FUNCTION "Gest Asse B Boxing" : VOID
TITLE =Gestione Asse B Boxing Rotazione Polso +90Gr/0Gr/-90Gr
AUTHOR : MassimoZ
FAMILY : NovaSrl
VERSION : 0.1

BEGIN
NETWORK
TITLE ======== PACO 1 =======

NETWORK
TITLE =INS./DISIN.1
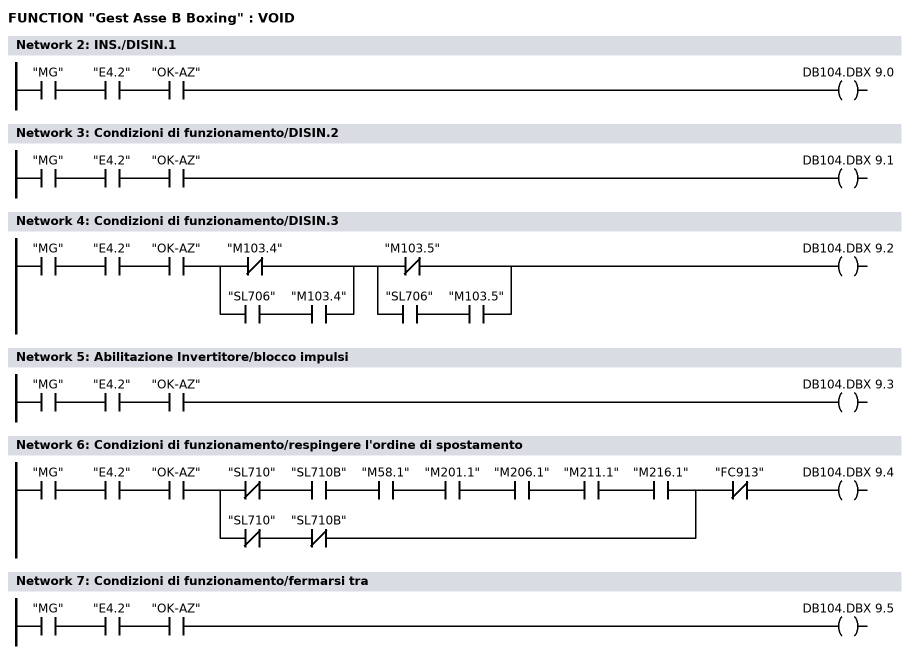
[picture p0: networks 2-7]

      U     "MG";
      U     "E4.2";
      U     "OK-AZ";
      =     DB104.DBX    9.0;
NETWORK
TITLE =Condizioni di funzionamento/DISIN.2

      U     "MG";
      U     "E4.2";
      U     "OK-AZ";
      =     DB104.DBX    9.1;
NETWORK
TITLE =Condizioni di funzionamento/DISIN.3

      U     "MG";
      U     "E4.2";
      U     "OK-AZ";
      U(    ;
      ON    "M103.4";
      O     ;
      U     "SL706";
      U     "M103.4";
      )     ;
      U(    ;
      ON    "M103.5";
      O     ;
      U     "SL706";
      U     "M103.5";
      )     ;
      =     DB104.DBX    9.2;
NETWORK
TITLE =Abilitazione Invertitore/blocco impulsi

      U     "MG";
      U     "E4.2";
      U     "OK-AZ";
      =     DB104.DBX    9.3;
NETWORK
TITLE =Condizioni di funzionamento/respingere l'ordine di spostamento

      U     "MG";
      U     "E4.2";
      U     "OK-AZ";
      U(    ;
      UN    "SL710";
      U     "SL710B";
      U     "M58.1";
      U     "M201.1";
      U     "M206.1";
      U     "M211.1";
      U     "M216.1";
      O     ;
      UN    "SL710";
      UN    "SL710B";
      )     ;
      UN    "FC913";
      =     DB104.DBX    9.4;
NETWORK
TITLE =Condizioni di funzionamento/fermarsi tra

      U     "MG";
      U     "E4.2";
      U     "OK-AZ";
      =     DB104.DBX    9.5;
NETWORK
TITLE =Attivare l'ordine di spostamento

      U(    ;
      U(    ;
      O     "M65.2";
      O     "M-ABPBS";
      O     "M+ABPBS";
      O     "M-ABPBD";
      O     "M+ABPBD";
      O     DB110.DBX    4.0;
      O     DB110.DBX    4.5;
      O     DB110.DBX    5.2;
      O     DB110.DBX    5.7;
      O     DB110.DBX    6.4;
      O     DB110.DBX    7.1;
      O     DB110.DBX   12.0;
      O     DB110.DBX   12.5;
      O     DB110.DBX   13.2;
      O     DB110.DBX   13.7;
      O     DB110.DBX   14.4;
      O     DB110.DBX   15.1;
      )     ;
      U(    ;
      UN    "SL710";
      U     "SL710B";
      O     ;
      UN    "SL710";
      UN    "SL710B";
      )     ;
      L     S5T#100MS;
      SE    T     52;
      NOP   0;
      NOP   0;
      NOP   0;
      U     T     52;
      )     ;
      FP    "M216.0";
      =     DB104.DBX    9.6;
NETWORK
TITLE =Reset memoria guasti
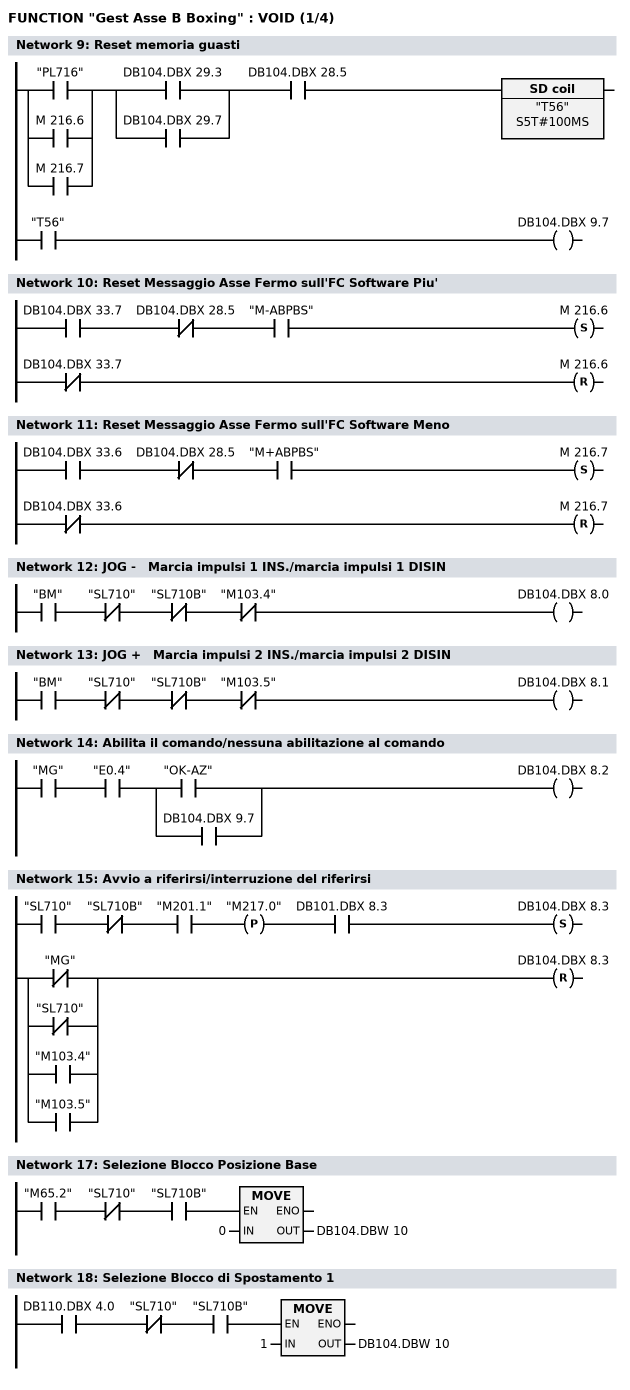
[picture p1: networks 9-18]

      U(    ;
      O     "PL716";
      O     M    216.6;
      O     M    216.7;
      )     ;
      U(    ;
      O     DB104.DBX   29.3;
      O     DB104.DBX   29.7;
      )     ;
      U     DB104.DBX   28.5;
      L     S5T#100MS;
      SE    "T56";
      NOP   0;
      NOP   0;
      NOP   0;
      U     "T56";
      =     DB104.DBX    9.7;
NETWORK
TITLE =Reset Messaggio Asse Fermo sull'FC Software Piu'

      U     DB104.DBX   33.7;
      UN    DB104.DBX   28.5;
      U     "M-ABPBS";
      S     M    216.6;
      UN    DB104.DBX   33.7;
      R     M    216.6;
      NOP   0;
NETWORK
TITLE =Reset Messaggio Asse Fermo sull'FC Software Meno

      U     DB104.DBX   33.6;
      UN    DB104.DBX   28.5;
      U     "M+ABPBS";
      S     M    216.7;
      UN    DB104.DBX   33.6;
      R     M    216.7;
      NOP   0;
NETWORK
TITLE =JOG -   Marcia impulsi 1 INS./marcia impulsi 1 DISIN

      U     "BM";
      UN    "SL710";
      UN    "SL710B";
      UN    "M103.4";
      =     DB104.DBX    8.0;
NETWORK
TITLE =JOG +   Marcia impulsi 2 INS./marcia impulsi 2 DISIN

      U     "BM";
      UN    "SL710";
      UN    "SL710B";
      UN    "M103.5";
      =     DB104.DBX    8.1;
NETWORK
TITLE =Abilita il comando/nessuna abilitazione al comando

      U     "MG";
      U     "E0.4";
      U(    ;
      O     "OK-AZ";
      O     DB104.DBX    9.7;
      )     ;
      =     DB104.DBX    8.2;
NETWORK
TITLE =Avvio a riferirsi/interruzione del riferirsi

      U     "SL710";
      UN    "SL710B";
      U     "M201.1";
      FP    "M217.0";
      U     DB101.DBX    8.3;
      S     DB104.DBX    8.3;
      U(    ;
      ON    "MG";
      ON    "SL710";
      O     "M103.4";
      O     "M103.5";
      )     ;
      R     DB104.DBX    8.3;
      NOP   0;
NETWORK
TITLE ======== SCELTA BLOCCO =======

NETWORK
TITLE =Selezione Blocco Posizione Base

      U     "M65.2";
      UN    "SL710";
      U     "SL710B";
      SPBNB _001;
      L     0;
      T     DB104.DBW   10;
_001: NOP   0;
NETWORK
TITLE =Selezione Blocco di Spostamento 1

      U     DB110.DBX    4.0;
      UN    "SL710";
      U     "SL710B";
      SPBNB _002;
      L     1;
      T     DB104.DBW   10;
_002: NOP   0;
NETWORK
TITLE =Selezione Blocco di Spostamento 2
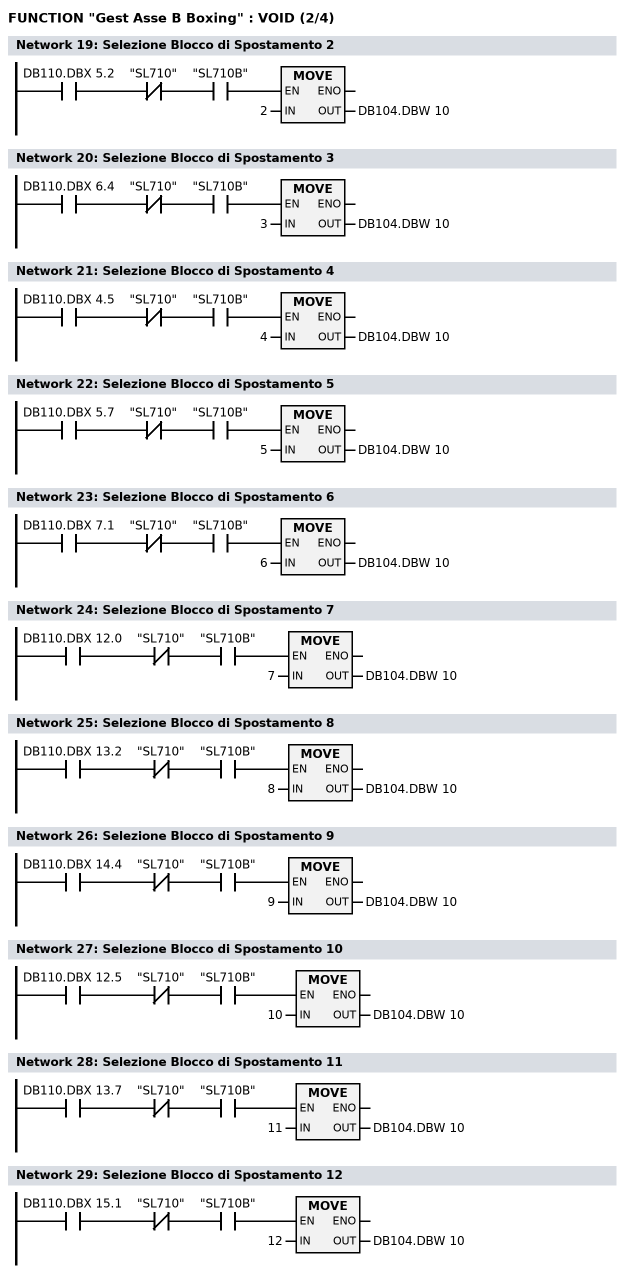
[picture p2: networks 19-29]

      U     DB110.DBX    5.2;
      UN    "SL710";
      U     "SL710B";
      SPBNB _003;
      L     2;
      T     DB104.DBW   10;
_003: NOP   0;
NETWORK
TITLE =Selezione Blocco di Spostamento 3

      U     DB110.DBX    6.4;
      UN    "SL710";
      U     "SL710B";
      SPBNB _004;
      L     3;
      T     DB104.DBW   10;
_004: NOP   0;
NETWORK
TITLE =Selezione Blocco di Spostamento 4

      U     DB110.DBX    4.5;
      UN    "SL710";
      U     "SL710B";
      SPBNB _005;
      L     4;
      T     DB104.DBW   10;
_005: NOP   0;
NETWORK
TITLE =Selezione Blocco di Spostamento 5

      U     DB110.DBX    5.7;
      UN    "SL710";
      U     "SL710B";
      SPBNB _006;
      L     5;
      T     DB104.DBW   10;
_006: NOP   0;
NETWORK
TITLE =Selezione Blocco di Spostamento 6

      U     DB110.DBX    7.1;
      UN    "SL710";
      U     "SL710B";
      SPBNB _007;
      L     6;
      T     DB104.DBW   10;
_007: NOP   0;
NETWORK
TITLE =Selezione Blocco di Spostamento 7

      U     DB110.DBX   12.0;
      UN    "SL710";
      U     "SL710B";
      SPBNB _008;
      L     7;
      T     DB104.DBW   10;
_008: NOP   0;
NETWORK
TITLE =Selezione Blocco di Spostamento 8

      U     DB110.DBX   13.2;
      UN    "SL710";
      U     "SL710B";
      SPBNB _009;
      L     8;
      T     DB104.DBW   10;
_009: NOP   0;
NETWORK
TITLE =Selezione Blocco di Spostamento 9

      U     DB110.DBX   14.4;
      UN    "SL710";
      U     "SL710B";
      SPBNB _00a;
      L     9;
      T     DB104.DBW   10;
_00a: NOP   0;
NETWORK
TITLE =Selezione Blocco di Spostamento 10

      U     DB110.DBX   12.5;
      UN    "SL710";
      U     "SL710B";
      SPBNB _00b;
      L     10;
      T     DB104.DBW   10;
_00b: NOP   0;
NETWORK
TITLE =Selezione Blocco di Spostamento 11

      U     DB110.DBX   13.7;
      UN    "SL710";
      U     "SL710B";
      SPBNB _00c;
      L     11;
      T     DB104.DBW   10;
_00c: NOP   0;
NETWORK
TITLE =Selezione Blocco di Spostamento 12

      U     DB110.DBX   15.1;
      UN    "SL710";
      U     "SL710B";
      SPBNB _00d;
      L     12;
      T     DB104.DBW   10;
_00d: NOP   0;
NETWORK
TITLE =Selezione Blocco di Spostamento 13 (0 Gradi Manuale)
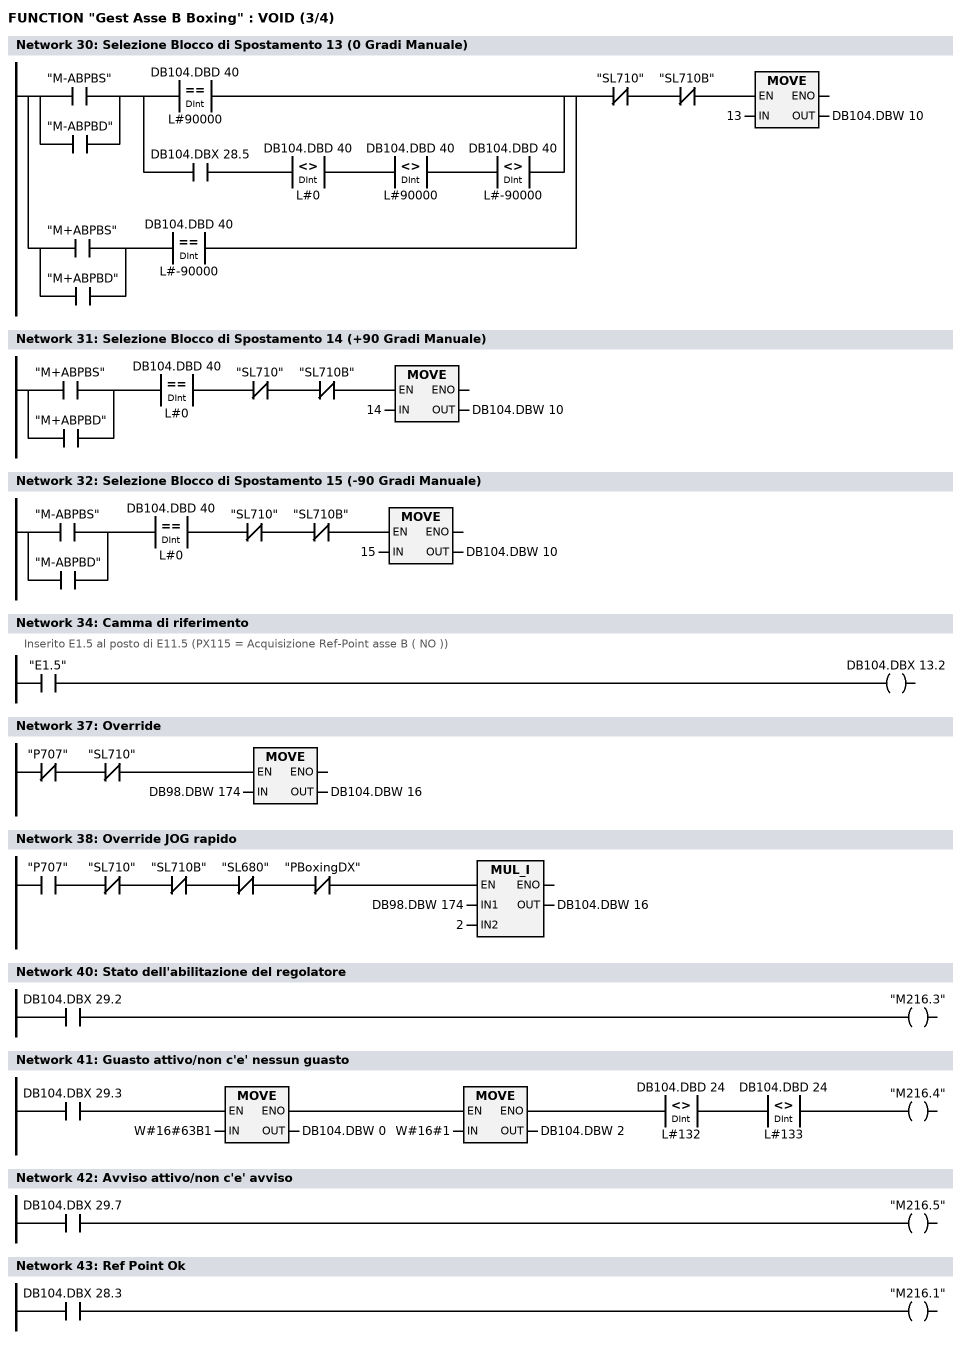
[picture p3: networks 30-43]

      U(    ;
      U(    ;
      O     "M-ABPBS";
      O     "M-ABPBD";
      )     ;
      U(    ;
      O(    ;
      L     DB104.DBD   40;
      L     L#90000;
      ==D   ;
      )     ;
      O     ;
      U     DB104.DBX   28.5;
      U(    ;
      L     DB104.DBD   40;
      L     L#0;
      <>D   ;
      )     ;
      U(    ;
      L     DB104.DBD   40;
      L     L#90000;
      <>D   ;
      )     ;
      U(    ;
      L     DB104.DBD   40;
      L     L#-90000;
      <>D   ;
      )     ;
      )     ;
      O     ;
      U(    ;
      O     "M+ABPBS";
      O     "M+ABPBD";
      )     ;
      U(    ;
      L     DB104.DBD   40;
      L     L#-90000;
      ==D   ;
      )     ;
      )     ;
      UN    "SL710";
      UN    "SL710B";
      SPBNB _00e;
      L     13;
      T     DB104.DBW   10;
_00e: NOP   0;
NETWORK
TITLE =Selezione Blocco di Spostamento 14 (+90 Gradi Manuale)

      U(    ;
      O     "M+ABPBS";
      O     "M+ABPBD";
      )     ;
      U(    ;
      L     DB104.DBD   40;
      L     L#0;
      ==D   ;
      )     ;
      UN    "SL710";
      UN    "SL710B";
      SPBNB _00f;
      L     14;
      T     DB104.DBW   10;
_00f: NOP   0;
NETWORK
TITLE =Selezione Blocco di Spostamento 15 (-90 Gradi Manuale)

      U(    ;
      O     "M-ABPBS";
      O     "M-ABPBD";
      )     ;
      U(    ;
      L     DB104.DBD   40;
      L     L#0;
      ==D   ;
      )     ;
      UN    "SL710";
      UN    "SL710B";
      SPBNB _010;
      L     15;
      T     DB104.DBW   10;
_010: NOP   0;
NETWORK
TITLE ======== POS PACO =======

NETWORK
TITLE =Camma di riferimento
//Inserito E1.5 al posto di E11.5 (PX115 = Acquisizione Ref-Point asse B ( NO ))
      U     "E1.5";
      =     DB104.DBX   13.2;
NETWORK
TITLE ======== PACO 2 ======= ( previsto )

NETWORK
TITLE ======== OVERRIDE ======

NETWORK
TITLE =Override

      UN    "P707";
      UN    "SL710";
      SPBNB _011;
      L     DB98.DBW  174;
      T     DB104.DBW   16;
_011: NOP   0;
NETWORK
TITLE =Override JOG rapido

      U     "P707";
      UN    "SL710";
      UN    "SL710B";
      UN    "SL680";
      UN    "PBoxingDX";
      SPBNB _012;
      L     DB98.DBW  174;
      L     2;
      *I    ;
      T     DB104.DBW   16;
_012: NOP   0;
NETWORK
TITLE ======== PAST 1 =======

NETWORK
TITLE =Stato dell'abilitazione del regolatore

      U     DB104.DBX   29.2;
      =     "M216.3";
NETWORK
TITLE =Guasto attivo/non c'e' nessun guasto

      U(    ;
      U(    ;
      U     DB104.DBX   29.3;
      SPBNB _013;
      L     W#16#63B1;
      T     DB104.DBW    0;
      SET   ;
      SAVE  ;
      CLR   ;
_013: U     BIE;
      )     ;
      SPBNB _014;
      L     W#16#1;
      T     DB104.DBW    2;
      SET   ;
      SAVE  ;
      CLR   ;
_014: U     BIE;
      )     ;
      U(    ;
      L     DB104.DBD   24;
      L     L#132;
      <>D   ;
      )     ;
      U(    ;
      L     DB104.DBD   24;
      L     L#133;
      <>D   ;
      )     ;
      =     "M216.4";
NETWORK
TITLE =Avviso attivo/non c'e' avviso

      U     DB104.DBX   29.7;
      =     "M216.5";
NETWORK
TITLE =Ref Point Ok

      U     DB104.DBX   28.3;
      =     "M216.1";
NETWORK
TITLE ======== POS PAST =======

NETWORK
TITLE ======== Lettura Quote =======

NETWORK
TITLE =Richiesta della Quota dell'asse B
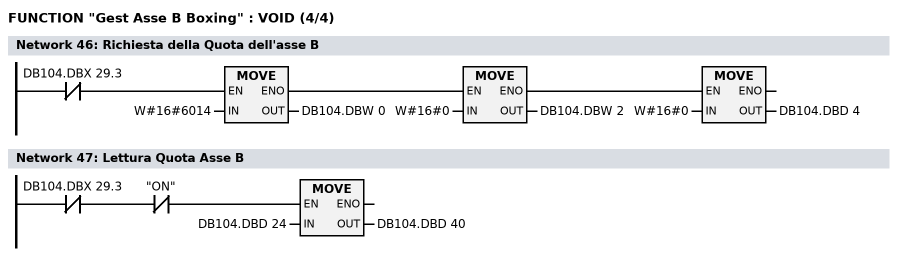
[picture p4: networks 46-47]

      U(    ;
      U(    ;
      UN    DB104.DBX   29.3;
      SPBNB _015;
      L     W#16#6014;
      T     DB104.DBW    0;
      SET   ;
      SAVE  ;
      CLR   ;
_015: U     BIE;
      )     ;
      SPBNB _016;
      L     W#16#0;
      T     DB104.DBW    2;
      SET   ;
      SAVE  ;
      CLR   ;
_016: U     BIE;
      )     ;
      SPBNB _017;
      L     W#16#0;
      T     DB104.DBD    4;
_017: NOP   0;
NETWORK
TITLE =Lettura Quota Asse B

      UN    DB104.DBX   29.3;
      UN    "ON";
      SPBNB _018;
      L     DB104.DBD   24;
      T     DB104.DBD   40;
_018: NOP   0;
NETWORK
TITLE ======== Caricamento quote sui Blocchi di Spostamento =======

NETWORK
TITLE =Caricamento Primo Posizionamento

      UN    "SL710";
      UN    "SL710B";
      U     DB99.DBX    3.3;
      O(    ;
      U     "MG";
      FP    M    254.4;
      )     ;
      O     "M219.0";
      =     L      0.0;
      U(    ;
      U(    ;
      U     L      0.0;
      UN    "M219.1";
      SPBNB _019;
      L     W#16#8051;
      T     DB104.DBW    0;
      SET   ;
      SAVE  ;
      CLR   ;
_019: U     BIE;
      )     ;
      SPBNB _01a;
      L     W#16#1;
      T     DB104.DBW    2;
      SET   ;
      SAVE  ;
      CLR   ;
_01a: U     BIE;
      )     ;
      SPBNB _01b;
      L     DB98.DBD  324;
      T     DB104.DBD    4;
_01b: NOP   0;
      U     L      0.0;
      BLD   102;
      S     "M219.0";
NETWORK
TITLE =Confronto Primo Posizionamento caricato nel 611U
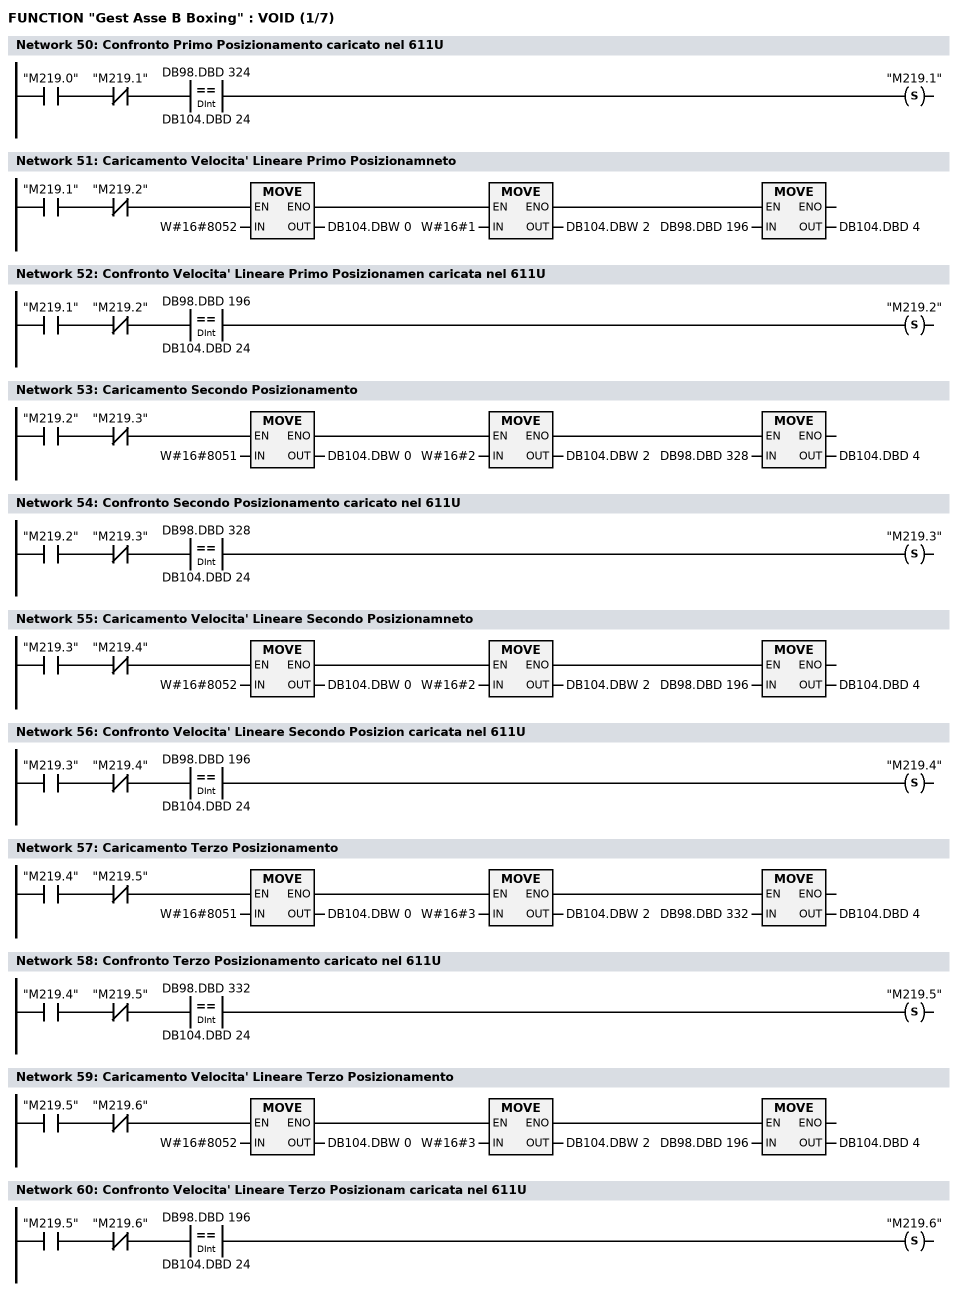
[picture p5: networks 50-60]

      U     "M219.0";
      UN    "M219.1";
      U(    ;
      L     DB98.DBD  324;
      L     DB104.DBD   24;
      ==D   ;
      )     ;
      S     "M219.1";
NETWORK
TITLE =Caricamento Velocita' Lineare Primo Posizionamneto

      U(    ;
      U(    ;
      U     "M219.1";
      UN    "M219.2";
      SPBNB _01c;
      L     W#16#8052;
      T     DB104.DBW    0;
      SET   ;
      SAVE  ;
      CLR   ;
_01c: U     BIE;
      )     ;
      SPBNB _01d;
      L     W#16#1;
      T     DB104.DBW    2;
      SET   ;
      SAVE  ;
      CLR   ;
_01d: U     BIE;
      )     ;
      SPBNB _01e;
      L     DB98.DBD  196;
      T     DB104.DBD    4;
_01e: NOP   0;
NETWORK
TITLE =Confronto Velocita' Lineare Primo Posizionamen caricata nel 611U

      U     "M219.1";
      UN    "M219.2";
      U(    ;
      L     DB98.DBD  196;
      L     DB104.DBD   24;
      ==D   ;
      )     ;
      S     "M219.2";
NETWORK
TITLE =Caricamento Secondo Posizionamento

      U(    ;
      U(    ;
      U     "M219.2";
      UN    "M219.3";
      SPBNB _01f;
      L     W#16#8051;
      T     DB104.DBW    0;
      SET   ;
      SAVE  ;
      CLR   ;
_01f: U     BIE;
      )     ;
      SPBNB _020;
      L     W#16#2;
      T     DB104.DBW    2;
      SET   ;
      SAVE  ;
      CLR   ;
_020: U     BIE;
      )     ;
      SPBNB _021;
      L     DB98.DBD  328;
      T     DB104.DBD    4;
_021: NOP   0;
NETWORK
TITLE =Confronto Secondo Posizionamento caricato nel 611U

      U     "M219.2";
      UN    "M219.3";
      U(    ;
      L     DB98.DBD  328;
      L     DB104.DBD   24;
      ==D   ;
      )     ;
      S     "M219.3";
NETWORK
TITLE =Caricamento Velocita' Lineare Secondo Posizionamneto

      U(    ;
      U(    ;
      U     "M219.3";
      UN    "M219.4";
      SPBNB _022;
      L     W#16#8052;
      T     DB104.DBW    0;
      SET   ;
      SAVE  ;
      CLR   ;
_022: U     BIE;
      )     ;
      SPBNB _023;
      L     W#16#2;
      T     DB104.DBW    2;
      SET   ;
      SAVE  ;
      CLR   ;
_023: U     BIE;
      )     ;
      SPBNB _024;
      L     DB98.DBD  196;
      T     DB104.DBD    4;
_024: NOP   0;
NETWORK
TITLE =Confronto Velocita' Lineare Secondo Posizion caricata nel 611U

      U     "M219.3";
      UN    "M219.4";
      U(    ;
      L     DB98.DBD  196;
      L     DB104.DBD   24;
      ==D   ;
      )     ;
      S     "M219.4";
NETWORK
TITLE =Caricamento Terzo Posizionamento

      U(    ;
      U(    ;
      U     "M219.4";
      UN    "M219.5";
      SPBNB _025;
      L     W#16#8051;
      T     DB104.DBW    0;
      SET   ;
      SAVE  ;
      CLR   ;
_025: U     BIE;
      )     ;
      SPBNB _026;
      L     W#16#3;
      T     DB104.DBW    2;
      SET   ;
      SAVE  ;
      CLR   ;
_026: U     BIE;
      )     ;
      SPBNB _027;
      L     DB98.DBD  332;
      T     DB104.DBD    4;
_027: NOP   0;
NETWORK
TITLE =Confronto Terzo Posizionamento caricato nel 611U

      U     "M219.4";
      UN    "M219.5";
      U(    ;
      L     DB98.DBD  332;
      L     DB104.DBD   24;
      ==D   ;
      )     ;
      S     "M219.5";
NETWORK
TITLE =Caricamento Velocita' Lineare Terzo Posizionamento

      U(    ;
      U(    ;
      U     "M219.5";
      UN    "M219.6";
      SPBNB _028;
      L     W#16#8052;
      T     DB104.DBW    0;
      SET   ;
      SAVE  ;
      CLR   ;
_028: U     BIE;
      )     ;
      SPBNB _029;
      L     W#16#3;
      T     DB104.DBW    2;
      SET   ;
      SAVE  ;
      CLR   ;
_029: U     BIE;
      )     ;
      SPBNB _02a;
      L     DB98.DBD  196;
      T     DB104.DBD    4;
_02a: NOP   0;
NETWORK
TITLE =Confronto Velocita' Lineare Terzo Posizionam caricata nel 611U

      U     "M219.5";
      UN    "M219.6";
      U(    ;
      L     DB98.DBD  196;
      L     DB104.DBD   24;
      ==D   ;
      )     ;
      S     "M219.6";
NETWORK
TITLE =Caricamento Quarto Posizionamento
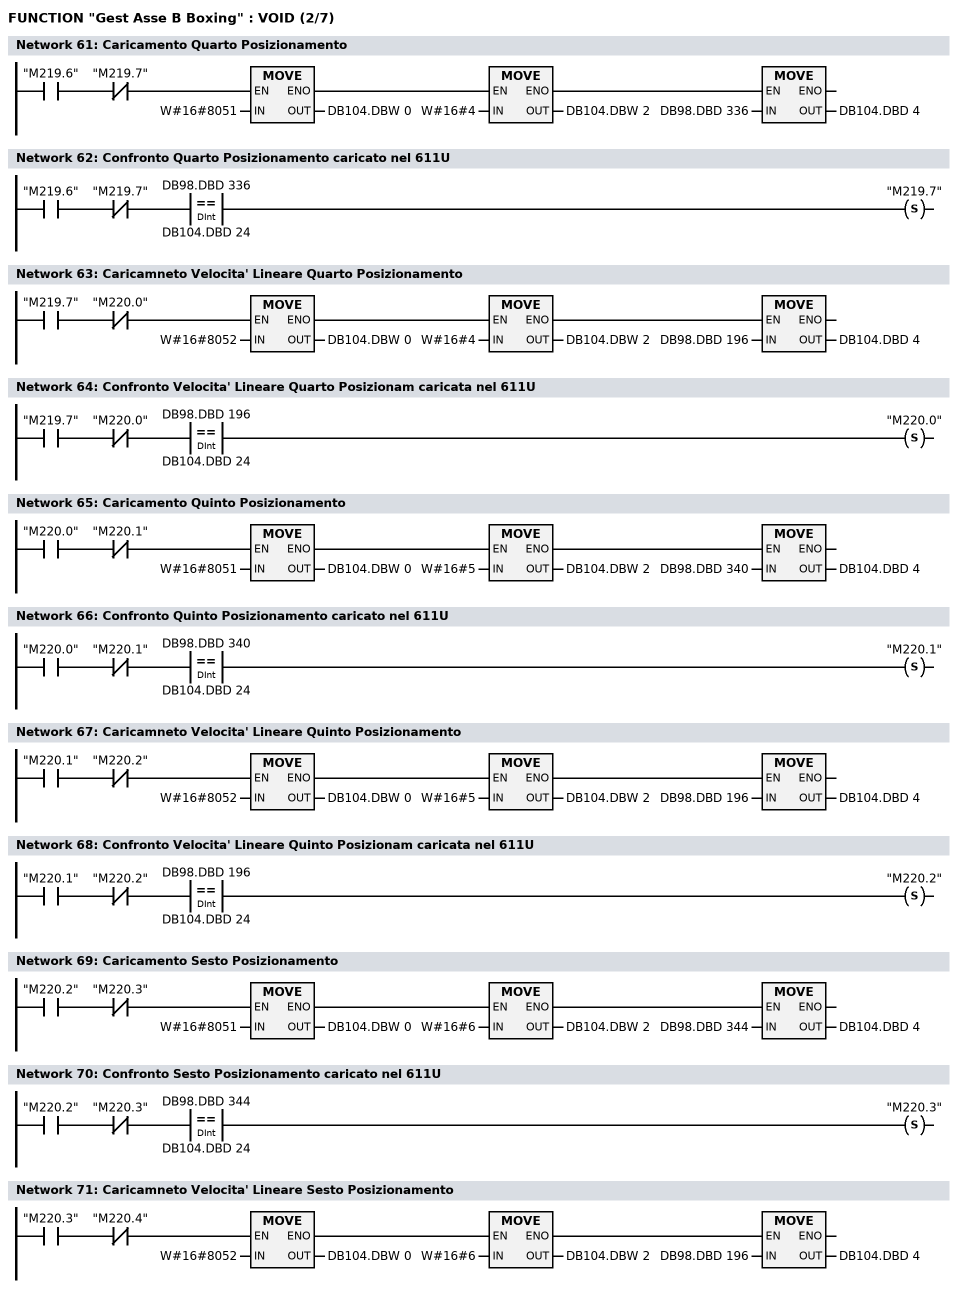
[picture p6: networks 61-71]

      U(    ;
      U(    ;
      U     "M219.6";
      UN    "M219.7";
      SPBNB _02b;
      L     W#16#8051;
      T     DB104.DBW    0;
      SET   ;
      SAVE  ;
      CLR   ;
_02b: U     BIE;
      )     ;
      SPBNB _02c;
      L     W#16#4;
      T     DB104.DBW    2;
      SET   ;
      SAVE  ;
      CLR   ;
_02c: U     BIE;
      )     ;
      SPBNB _02d;
      L     DB98.DBD  336;
      T     DB104.DBD    4;
_02d: NOP   0;
NETWORK
TITLE =Confronto Quarto Posizionamento caricato nel 611U

      U     "M219.6";
      UN    "M219.7";
      U(    ;
      L     DB98.DBD  336;
      L     DB104.DBD   24;
      ==D   ;
      )     ;
      S     "M219.7";
NETWORK
TITLE =Caricamneto Velocita' Lineare Quarto Posizionamento

      U(    ;
      U(    ;
      U     "M219.7";
      UN    "M220.0";
      SPBNB _02e;
      L     W#16#8052;
      T     DB104.DBW    0;
      SET   ;
      SAVE  ;
      CLR   ;
_02e: U     BIE;
      )     ;
      SPBNB _02f;
      L     W#16#4;
      T     DB104.DBW    2;
      SET   ;
      SAVE  ;
      CLR   ;
_02f: U     BIE;
      )     ;
      SPBNB _030;
      L     DB98.DBD  196;
      T     DB104.DBD    4;
_030: NOP   0;
NETWORK
TITLE =Confronto Velocita' Lineare Quarto Posizionam caricata nel 611U

      U     "M219.7";
      UN    "M220.0";
      U(    ;
      L     DB98.DBD  196;
      L     DB104.DBD   24;
      ==D   ;
      )     ;
      S     "M220.0";
NETWORK
TITLE =Caricamento Quinto Posizionamento

      U(    ;
      U(    ;
      U     "M220.0";
      UN    "M220.1";
      SPBNB _031;
      L     W#16#8051;
      T     DB104.DBW    0;
      SET   ;
      SAVE  ;
      CLR   ;
_031: U     BIE;
      )     ;
      SPBNB _032;
      L     W#16#5;
      T     DB104.DBW    2;
      SET   ;
      SAVE  ;
      CLR   ;
_032: U     BIE;
      )     ;
      SPBNB _033;
      L     DB98.DBD  340;
      T     DB104.DBD    4;
_033: NOP   0;
NETWORK
TITLE =Confronto Quinto Posizionamento caricato nel 611U

      U     "M220.0";
      UN    "M220.1";
      U(    ;
      L     DB98.DBD  340;
      L     DB104.DBD   24;
      ==D   ;
      )     ;
      S     "M220.1";
NETWORK
TITLE =Caricamneto Velocita' Lineare Quinto Posizionamento

      U(    ;
      U(    ;
      U     "M220.1";
      UN    "M220.2";
      SPBNB _034;
      L     W#16#8052;
      T     DB104.DBW    0;
      SET   ;
      SAVE  ;
      CLR   ;
_034: U     BIE;
      )     ;
      SPBNB _035;
      L     W#16#5;
      T     DB104.DBW    2;
      SET   ;
      SAVE  ;
      CLR   ;
_035: U     BIE;
      )     ;
      SPBNB _036;
      L     DB98.DBD  196;
      T     DB104.DBD    4;
_036: NOP   0;
NETWORK
TITLE =Confronto Velocita' Lineare Quinto Posizionam caricata nel 611U

      U     "M220.1";
      UN    "M220.2";
      U(    ;
      L     DB98.DBD  196;
      L     DB104.DBD   24;
      ==D   ;
      )     ;
      S     "M220.2";
NETWORK
TITLE =Caricamento Sesto Posizionamento

      U(    ;
      U(    ;
      U     "M220.2";
      UN    "M220.3";
      SPBNB _037;
      L     W#16#8051;
      T     DB104.DBW    0;
      SET   ;
      SAVE  ;
      CLR   ;
_037: U     BIE;
      )     ;
      SPBNB _038;
      L     W#16#6;
      T     DB104.DBW    2;
      SET   ;
      SAVE  ;
      CLR   ;
_038: U     BIE;
      )     ;
      SPBNB _039;
      L     DB98.DBD  344;
      T     DB104.DBD    4;
_039: NOP   0;
NETWORK
TITLE =Confronto Sesto Posizionamento caricato nel 611U

      U     "M220.2";
      UN    "M220.3";
      U(    ;
      L     DB98.DBD  344;
      L     DB104.DBD   24;
      ==D   ;
      )     ;
      S     "M220.3";
NETWORK
TITLE =Caricamneto Velocita' Lineare Sesto Posizionamento

      U(    ;
      U(    ;
      U     "M220.3";
      UN    "M220.4";
      SPBNB _03a;
      L     W#16#8052;
      T     DB104.DBW    0;
      SET   ;
      SAVE  ;
      CLR   ;
_03a: U     BIE;
      )     ;
      SPBNB _03b;
      L     W#16#6;
      T     DB104.DBW    2;
      SET   ;
      SAVE  ;
      CLR   ;
_03b: U     BIE;
      )     ;
      SPBNB _03c;
      L     DB98.DBD  196;
      T     DB104.DBD    4;
_03c: NOP   0;
NETWORK
TITLE =Confronto Velocita' Lineare Sesto Posizionam caricata nel 611U
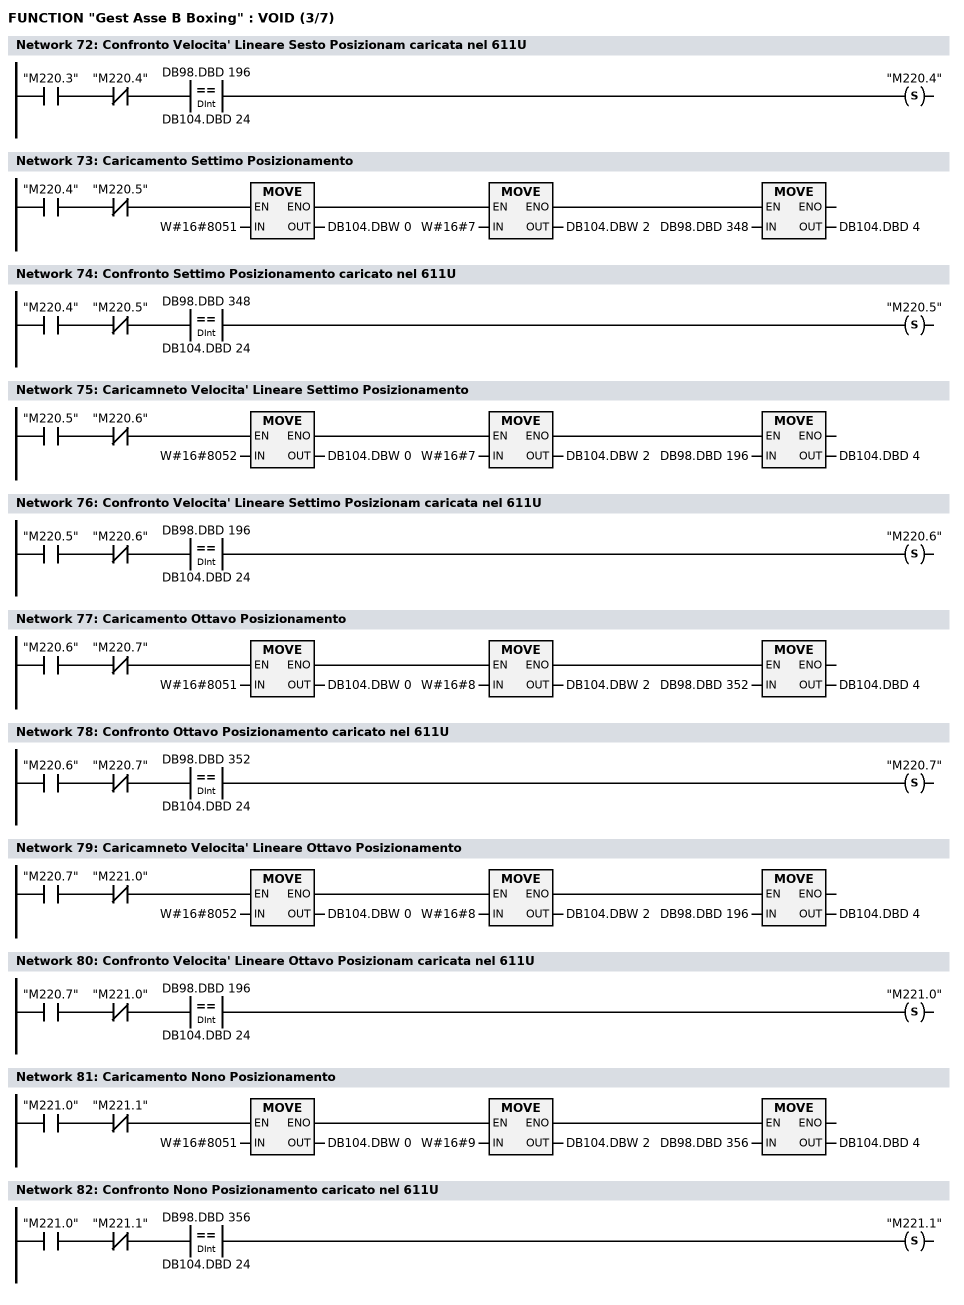
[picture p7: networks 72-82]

      U     "M220.3";
      UN    "M220.4";
      U(    ;
      L     DB98.DBD  196;
      L     DB104.DBD   24;
      ==D   ;
      )     ;
      S     "M220.4";
NETWORK
TITLE =Caricamento Settimo Posizionamento

      U(    ;
      U(    ;
      U     "M220.4";
      UN    "M220.5";
      SPBNB _03d;
      L     W#16#8051;
      T     DB104.DBW    0;
      SET   ;
      SAVE  ;
      CLR   ;
_03d: U     BIE;
      )     ;
      SPBNB _03e;
      L     W#16#7;
      T     DB104.DBW    2;
      SET   ;
      SAVE  ;
      CLR   ;
_03e: U     BIE;
      )     ;
      SPBNB _03f;
      L     DB98.DBD  348;
      T     DB104.DBD    4;
_03f: NOP   0;
NETWORK
TITLE =Confronto Settimo Posizionamento caricato nel 611U

      U     "M220.4";
      UN    "M220.5";
      U(    ;
      L     DB98.DBD  348;
      L     DB104.DBD   24;
      ==D   ;
      )     ;
      S     "M220.5";
NETWORK
TITLE =Caricamneto Velocita' Lineare Settimo Posizionamento

      U(    ;
      U(    ;
      U     "M220.5";
      UN    "M220.6";
      SPBNB _040;
      L     W#16#8052;
      T     DB104.DBW    0;
      SET   ;
      SAVE  ;
      CLR   ;
_040: U     BIE;
      )     ;
      SPBNB _041;
      L     W#16#7;
      T     DB104.DBW    2;
      SET   ;
      SAVE  ;
      CLR   ;
_041: U     BIE;
      )     ;
      SPBNB _042;
      L     DB98.DBD  196;
      T     DB104.DBD    4;
_042: NOP   0;
NETWORK
TITLE =Confronto Velocita' Lineare Settimo Posizionam caricata nel 611U

      U     "M220.5";
      UN    "M220.6";
      U(    ;
      L     DB98.DBD  196;
      L     DB104.DBD   24;
      ==D   ;
      )     ;
      S     "M220.6";
NETWORK
TITLE =Caricamento Ottavo Posizionamento

      U(    ;
      U(    ;
      U     "M220.6";
      UN    "M220.7";
      SPBNB _043;
      L     W#16#8051;
      T     DB104.DBW    0;
      SET   ;
      SAVE  ;
      CLR   ;
_043: U     BIE;
      )     ;
      SPBNB _044;
      L     W#16#8;
      T     DB104.DBW    2;
      SET   ;
      SAVE  ;
      CLR   ;
_044: U     BIE;
      )     ;
      SPBNB _045;
      L     DB98.DBD  352;
      T     DB104.DBD    4;
_045: NOP   0;
NETWORK
TITLE =Confronto Ottavo Posizionamento caricato nel 611U

      U     "M220.6";
      UN    "M220.7";
      U(    ;
      L     DB98.DBD  352;
      L     DB104.DBD   24;
      ==D   ;
      )     ;
      S     "M220.7";
NETWORK
TITLE =Caricamneto Velocita' Lineare Ottavo Posizionamento

      U(    ;
      U(    ;
      U     "M220.7";
      UN    "M221.0";
      SPBNB _046;
      L     W#16#8052;
      T     DB104.DBW    0;
      SET   ;
      SAVE  ;
      CLR   ;
_046: U     BIE;
      )     ;
      SPBNB _047;
      L     W#16#8;
      T     DB104.DBW    2;
      SET   ;
      SAVE  ;
      CLR   ;
_047: U     BIE;
      )     ;
      SPBNB _048;
      L     DB98.DBD  196;
      T     DB104.DBD    4;
_048: NOP   0;
NETWORK
TITLE =Confronto Velocita' Lineare Ottavo Posizionam caricata nel 611U

      U     "M220.7";
      UN    "M221.0";
      U(    ;
      L     DB98.DBD  196;
      L     DB104.DBD   24;
      ==D   ;
      )     ;
      S     "M221.0";
NETWORK
TITLE =Caricamento Nono Posizionamento

      U(    ;
      U(    ;
      U     "M221.0";
      UN    "M221.1";
      SPBNB _049;
      L     W#16#8051;
      T     DB104.DBW    0;
      SET   ;
      SAVE  ;
      CLR   ;
_049: U     BIE;
      )     ;
      SPBNB _04a;
      L     W#16#9;
      T     DB104.DBW    2;
      SET   ;
      SAVE  ;
      CLR   ;
_04a: U     BIE;
      )     ;
      SPBNB _04b;
      L     DB98.DBD  356;
      T     DB104.DBD    4;
_04b: NOP   0;
NETWORK
TITLE =Confronto Nono Posizionamento caricato nel 611U

      U     "M221.0";
      UN    "M221.1";
      U(    ;
      L     DB98.DBD  356;
      L     DB104.DBD   24;
      ==D   ;
      )     ;
      S     "M221.1";
NETWORK
TITLE =Caricamneto Velocita' Lineare Nono Posizionamento
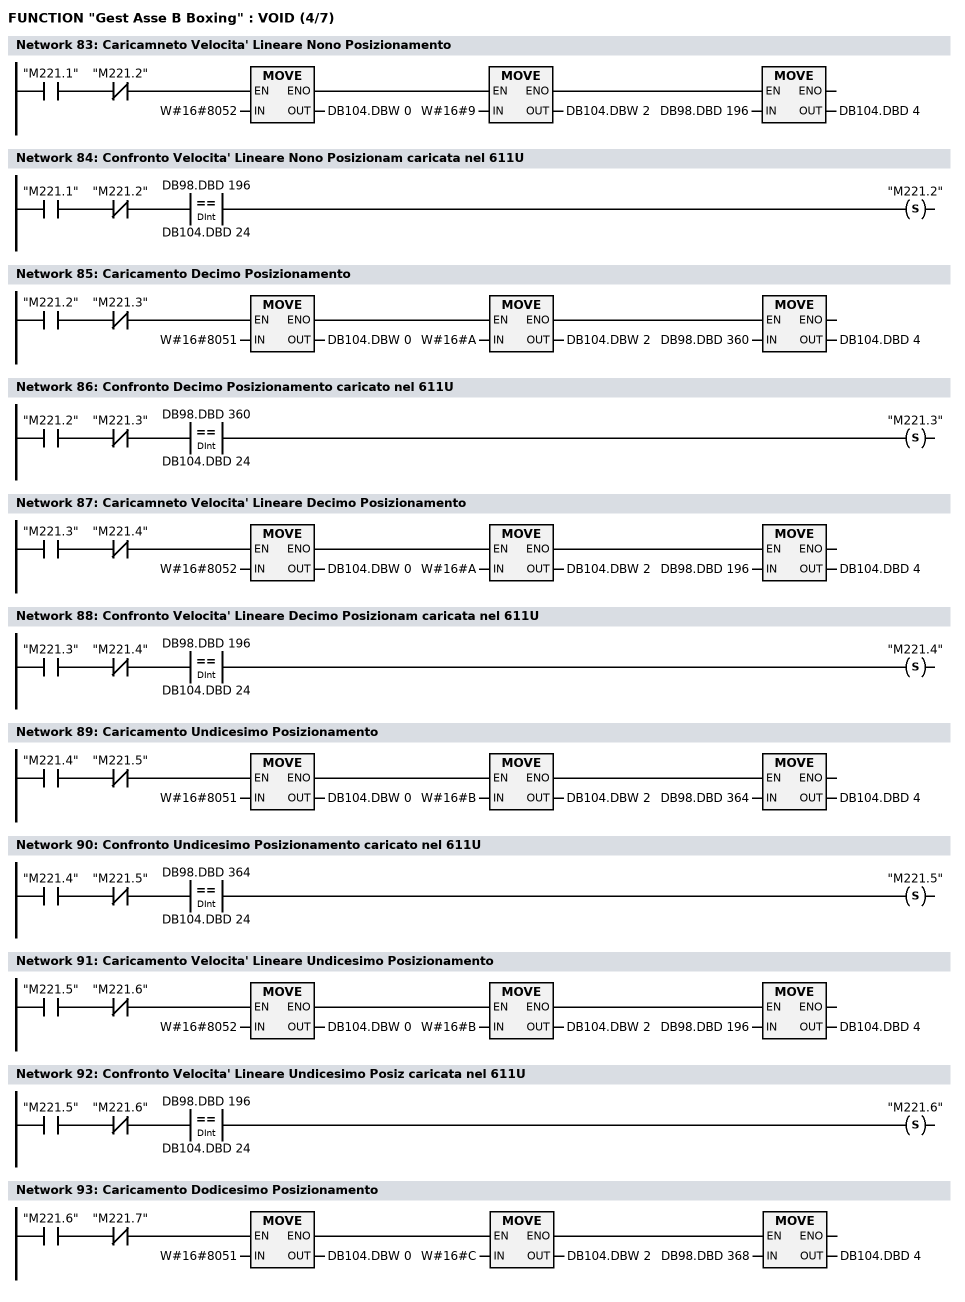
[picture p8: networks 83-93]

      U(    ;
      U(    ;
      U     "M221.1";
      UN    "M221.2";
      SPBNB _04c;
      L     W#16#8052;
      T     DB104.DBW    0;
      SET   ;
      SAVE  ;
      CLR   ;
_04c: U     BIE;
      )     ;
      SPBNB _04d;
      L     W#16#9;
      T     DB104.DBW    2;
      SET   ;
      SAVE  ;
      CLR   ;
_04d: U     BIE;
      )     ;
      SPBNB _04e;
      L     DB98.DBD  196;
      T     DB104.DBD    4;
_04e: NOP   0;
NETWORK
TITLE =Confronto Velocita' Lineare Nono Posizionam caricata nel 611U

      U     "M221.1";
      UN    "M221.2";
      U(    ;
      L     DB98.DBD  196;
      L     DB104.DBD   24;
      ==D   ;
      )     ;
      S     "M221.2";
NETWORK
TITLE =Caricamento Decimo Posizionamento

      U(    ;
      U(    ;
      U     "M221.2";
      UN    "M221.3";
      SPBNB _04f;
      L     W#16#8051;
      T     DB104.DBW    0;
      SET   ;
      SAVE  ;
      CLR   ;
_04f: U     BIE;
      )     ;
      SPBNB _050;
      L     W#16#A;
      T     DB104.DBW    2;
      SET   ;
      SAVE  ;
      CLR   ;
_050: U     BIE;
      )     ;
      SPBNB _051;
      L     DB98.DBD  360;
      T     DB104.DBD    4;
_051: NOP   0;
NETWORK
TITLE =Confronto Decimo Posizionamento caricato nel 611U

      U     "M221.2";
      UN    "M221.3";
      U(    ;
      L     DB98.DBD  360;
      L     DB104.DBD   24;
      ==D   ;
      )     ;
      S     "M221.3";
NETWORK
TITLE =Caricamneto Velocita' Lineare Decimo Posizionamento

      U(    ;
      U(    ;
      U     "M221.3";
      UN    "M221.4";
      SPBNB _052;
      L     W#16#8052;
      T     DB104.DBW    0;
      SET   ;
      SAVE  ;
      CLR   ;
_052: U     BIE;
      )     ;
      SPBNB _053;
      L     W#16#A;
      T     DB104.DBW    2;
      SET   ;
      SAVE  ;
      CLR   ;
_053: U     BIE;
      )     ;
      SPBNB _054;
      L     DB98.DBD  196;
      T     DB104.DBD    4;
_054: NOP   0;
NETWORK
TITLE =Confronto Velocita' Lineare Decimo Posizionam caricata nel 611U

      U     "M221.3";
      UN    "M221.4";
      U(    ;
      L     DB98.DBD  196;
      L     DB104.DBD   24;
      ==D   ;
      )     ;
      S     "M221.4";
NETWORK
TITLE =Caricamento Undicesimo Posizionamento

      U(    ;
      U(    ;
      U     "M221.4";
      UN    "M221.5";
      SPBNB _055;
      L     W#16#8051;
      T     DB104.DBW    0;
      SET   ;
      SAVE  ;
      CLR   ;
_055: U     BIE;
      )     ;
      SPBNB _056;
      L     W#16#B;
      T     DB104.DBW    2;
      SET   ;
      SAVE  ;
      CLR   ;
_056: U     BIE;
      )     ;
      SPBNB _057;
      L     DB98.DBD  364;
      T     DB104.DBD    4;
_057: NOP   0;
NETWORK
TITLE =Confronto Undicesimo Posizionamento caricato nel 611U

      U     "M221.4";
      UN    "M221.5";
      U(    ;
      L     DB98.DBD  364;
      L     DB104.DBD   24;
      ==D   ;
      )     ;
      S     "M221.5";
NETWORK
TITLE =Caricamento Velocita' Lineare Undicesimo Posizionamento

      U(    ;
      U(    ;
      U     "M221.5";
      UN    "M221.6";
      SPBNB _058;
      L     W#16#8052;
      T     DB104.DBW    0;
      SET   ;
      SAVE  ;
      CLR   ;
_058: U     BIE;
      )     ;
      SPBNB _059;
      L     W#16#B;
      T     DB104.DBW    2;
      SET   ;
      SAVE  ;
      CLR   ;
_059: U     BIE;
      )     ;
      SPBNB _05a;
      L     DB98.DBD  196;
      T     DB104.DBD    4;
_05a: NOP   0;
NETWORK
TITLE =Confronto Velocita' Lineare Undicesimo Posiz caricata nel 611U

      U     "M221.5";
      UN    "M221.6";
      U(    ;
      L     DB98.DBD  196;
      L     DB104.DBD   24;
      ==D   ;
      )     ;
      S     "M221.6";
NETWORK
TITLE =Caricamento Dodicesimo Posizionamento

      U(    ;
      U(    ;
      U     "M221.6";
      UN    "M221.7";
      SPBNB _05b;
      L     W#16#8051;
      T     DB104.DBW    0;
      SET   ;
      SAVE  ;
      CLR   ;
_05b: U     BIE;
      )     ;
      SPBNB _05c;
      L     W#16#C;
      T     DB104.DBW    2;
      SET   ;
      SAVE  ;
      CLR   ;
_05c: U     BIE;
      )     ;
      SPBNB _05d;
      L     DB98.DBD  368;
      T     DB104.DBD    4;
_05d: NOP   0;
NETWORK
TITLE =Confronto Dodicesimo Posizionamento caricato nel 611U
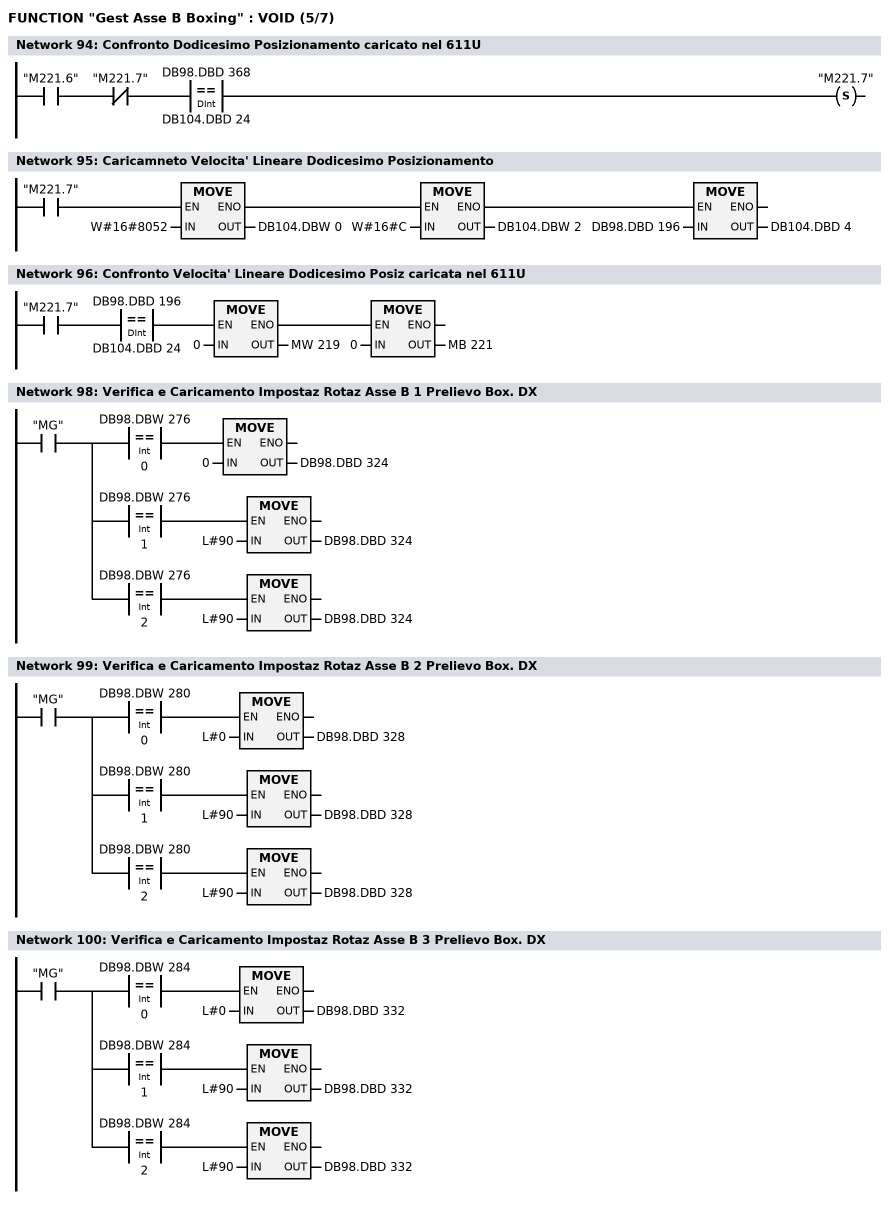
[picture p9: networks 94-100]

      U     "M221.6";
      UN    "M221.7";
      U(    ;
      L     DB98.DBD  368;
      L     DB104.DBD   24;
      ==D   ;
      )     ;
      S     "M221.7";
NETWORK
TITLE =Caricamneto Velocita' Lineare Dodicesimo Posizionamento

      U(    ;
      U(    ;
      U     "M221.7";
      SPBNB _05e;
      L     W#16#8052;
      T     DB104.DBW    0;
      SET   ;
      SAVE  ;
      CLR   ;
_05e: U     BIE;
      )     ;
      SPBNB _05f;
      L     W#16#C;
      T     DB104.DBW    2;
      SET   ;
      SAVE  ;
      CLR   ;
_05f: U     BIE;
      )     ;
      SPBNB _060;
      L     DB98.DBD  196;
      T     DB104.DBD    4;
_060: NOP   0;
NETWORK
TITLE =Confronto Velocita' Lineare Dodicesimo Posiz caricata nel 611U

      U(    ;
      U     "M221.7";
      U(    ;
      L     DB98.DBD  196;
      L     DB104.DBD   24;
      ==D   ;
      )     ;
      SPBNB _061;
      L     0;
      T     MW   219;
      SET   ;
      SAVE  ;
      CLR   ;
_061: U     BIE;
      )     ;
      SPBNB _062;
      L     0;
      T     MB   221;
_062: NOP   0;
NETWORK
TITLE ======== Caricamento Softkey OP sulle DB delle Quote Asse B =====

NETWORK
TITLE =Verifica e Caricamento Impostaz Rotaz Asse B 1 Prelievo Box. DX

      U     "MG";
      =     L      0.0;
      U     L      0.0;
      U(    ;
      L     DB98.DBW  276;
      L     0;
      ==I   ;
      )     ;
      SPBNB _063;
      L     0;
      T     DB98.DBD  324;
_063: NOP   0;
      U     L      0.0;
      U(    ;
      L     DB98.DBW  276;
      L     1;
      ==I   ;
      )     ;
      SPBNB _064;
      L     L#90;
      T     DB98.DBD  324;
_064: NOP   0;
      U     L      0.0;
      U(    ;
      L     DB98.DBW  276;
      L     2;
      ==I   ;
      )     ;
      SPBNB _065;
      L     L#90;
      T     DB98.DBD  324;
_065: NOP   0;
NETWORK
TITLE =Verifica e Caricamento Impostaz Rotaz Asse B 2 Prelievo Box. DX

      U     "MG";
      =     L      0.0;
      U     L      0.0;
      U(    ;
      L     DB98.DBW  280;
      L     0;
      ==I   ;
      )     ;
      SPBNB _066;
      L     L#0;
      T     DB98.DBD  328;
_066: NOP   0;
      U     L      0.0;
      U(    ;
      L     DB98.DBW  280;
      L     1;
      ==I   ;
      )     ;
      SPBNB _067;
      L     L#90;
      T     DB98.DBD  328;
_067: NOP   0;
      U     L      0.0;
      U(    ;
      L     DB98.DBW  280;
      L     2;
      ==I   ;
      )     ;
      SPBNB _068;
      L     L#90;
      T     DB98.DBD  328;
_068: NOP   0;
NETWORK
TITLE =Verifica e Caricamento Impostaz Rotaz Asse B 3 Prelievo Box. DX

      U     "MG";
      =     L      0.0;
      U     L      0.0;
      U(    ;
      L     DB98.DBW  284;
      L     0;
      ==I   ;
      )     ;
      SPBNB _069;
      L     L#0;
      T     DB98.DBD  332;
_069: NOP   0;
      U     L      0.0;
      U(    ;
      L     DB98.DBW  284;
      L     1;
      ==I   ;
      )     ;
      SPBNB _06a;
      L     L#90;
      T     DB98.DBD  332;
_06a: NOP   0;
      U     L      0.0;
      U(    ;
      L     DB98.DBW  284;
      L     2;
      ==I   ;
      )     ;
      SPBNB _06b;
      L     L#90;
      T     DB98.DBD  332;
_06b: NOP   0;
NETWORK
TITLE =Verifica e Caricamento Impostaz Rotaz Asse B 1 Deposito Box. DX
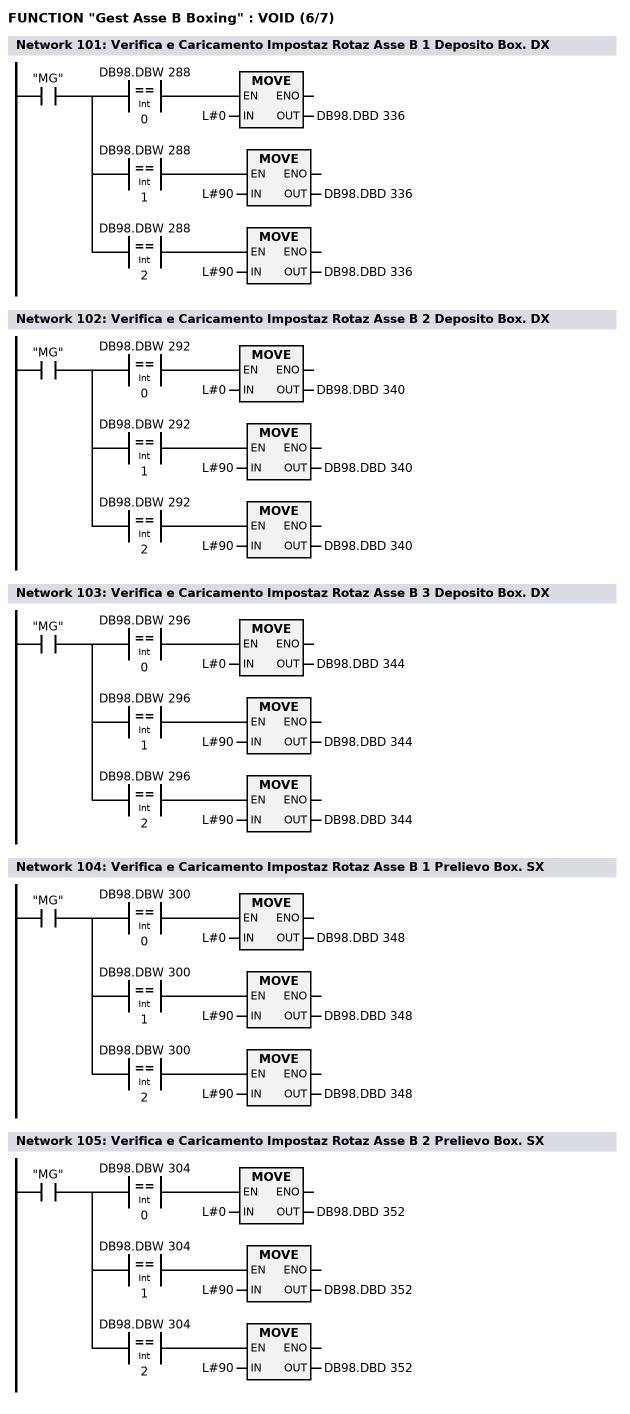
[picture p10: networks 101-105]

      U     "MG";
      =     L      0.0;
      U     L      0.0;
      U(    ;
      L     DB98.DBW  288;
      L     0;
      ==I   ;
      )     ;
      SPBNB _06c;
      L     L#0;
      T     DB98.DBD  336;
_06c: NOP   0;
      U     L      0.0;
      U(    ;
      L     DB98.DBW  288;
      L     1;
      ==I   ;
      )     ;
      SPBNB _06d;
      L     L#90;
      T     DB98.DBD  336;
_06d: NOP   0;
      U     L      0.0;
      U(    ;
      L     DB98.DBW  288;
      L     2;
      ==I   ;
      )     ;
      SPBNB _06e;
      L     L#90;
      T     DB98.DBD  336;
_06e: NOP   0;
NETWORK
TITLE =Verifica e Caricamento Impostaz Rotaz Asse B 2 Deposito Box. DX

      U     "MG";
      =     L      0.0;
      U     L      0.0;
      U(    ;
      L     DB98.DBW  292;
      L     0;
      ==I   ;
      )     ;
      SPBNB _06f;
      L     L#0;
      T     DB98.DBD  340;
_06f: NOP   0;
      U     L      0.0;
      U(    ;
      L     DB98.DBW  292;
      L     1;
      ==I   ;
      )     ;
      SPBNB _070;
      L     L#90;
      T     DB98.DBD  340;
_070: NOP   0;
      U     L      0.0;
      U(    ;
      L     DB98.DBW  292;
      L     2;
      ==I   ;
      )     ;
      SPBNB _071;
      L     L#90;
      T     DB98.DBD  340;
_071: NOP   0;
NETWORK
TITLE =Verifica e Caricamento Impostaz Rotaz Asse B 3 Deposito Box. DX

      U     "MG";
      =     L      0.0;
      U     L      0.0;
      U(    ;
      L     DB98.DBW  296;
      L     0;
      ==I   ;
      )     ;
      SPBNB _072;
      L     L#0;
      T     DB98.DBD  344;
_072: NOP   0;
      U     L      0.0;
      U(    ;
      L     DB98.DBW  296;
      L     1;
      ==I   ;
      )     ;
      SPBNB _073;
      L     L#90;
      T     DB98.DBD  344;
_073: NOP   0;
      U     L      0.0;
      U(    ;
      L     DB98.DBW  296;
      L     2;
      ==I   ;
      )     ;
      SPBNB _074;
      L     L#90;
      T     DB98.DBD  344;
_074: NOP   0;
NETWORK
TITLE =Verifica e Caricamento Impostaz Rotaz Asse B 1 Prelievo Box. SX

      U     "MG";
      =     L      0.0;
      U     L      0.0;
      U(    ;
      L     DB98.DBW  300;
      L     0;
      ==I   ;
      )     ;
      SPBNB _075;
      L     L#0;
      T     DB98.DBD  348;
_075: NOP   0;
      U     L      0.0;
      U(    ;
      L     DB98.DBW  300;
      L     1;
      ==I   ;
      )     ;
      SPBNB _076;
      L     L#90;
      T     DB98.DBD  348;
_076: NOP   0;
      U     L      0.0;
      U(    ;
      L     DB98.DBW  300;
      L     2;
      ==I   ;
      )     ;
      SPBNB _077;
      L     L#90;
      T     DB98.DBD  348;
_077: NOP   0;
NETWORK
TITLE =Verifica e Caricamento Impostaz Rotaz Asse B 2 Prelievo Box. SX

      U     "MG";
      =     L      0.0;
      U     L      0.0;
      U(    ;
      L     DB98.DBW  304;
      L     0;
      ==I   ;
      )     ;
      SPBNB _078;
      L     L#0;
      T     DB98.DBD  352;
_078: NOP   0;
      U     L      0.0;
      U(    ;
      L     DB98.DBW  304;
      L     1;
      ==I   ;
      )     ;
      SPBNB _079;
      L     L#90;
      T     DB98.DBD  352;
_079: NOP   0;
      U     L      0.0;
      U(    ;
      L     DB98.DBW  304;
      L     2;
      ==I   ;
      )     ;
      SPBNB _07a;
      L     L#90;
      T     DB98.DBD  352;
_07a: NOP   0;
NETWORK
TITLE =Verifica e Caricamento Impostaz Rotaz Asse B 3 Prelievo Box. SX
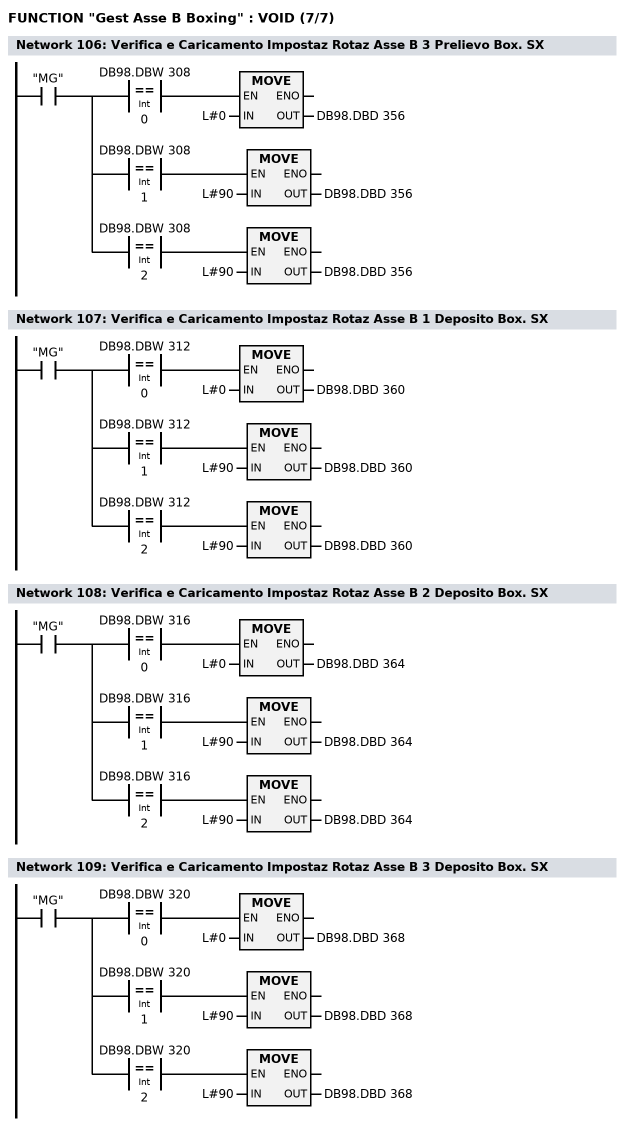
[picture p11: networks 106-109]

      U     "MG";
      =     L      0.0;
      U     L      0.0;
      U(    ;
      L     DB98.DBW  308;
      L     0;
      ==I   ;
      )     ;
      SPBNB _07b;
      L     L#0;
      T     DB98.DBD  356;
_07b: NOP   0;
      U     L      0.0;
      U(    ;
      L     DB98.DBW  308;
      L     1;
      ==I   ;
      )     ;
      SPBNB _07c;
      L     L#90;
      T     DB98.DBD  356;
_07c: NOP   0;
      U     L      0.0;
      U(    ;
      L     DB98.DBW  308;
      L     2;
      ==I   ;
      )     ;
      SPBNB _07d;
      L     L#90;
      T     DB98.DBD  356;
_07d: NOP   0;
NETWORK
TITLE =Verifica e Caricamento Impostaz Rotaz Asse B 1 Deposito Box. SX

      U     "MG";
      =     L      0.0;
      U     L      0.0;
      U(    ;
      L     DB98.DBW  312;
      L     0;
      ==I   ;
      )     ;
      SPBNB _07e;
      L     L#0;
      T     DB98.DBD  360;
_07e: NOP   0;
      U     L      0.0;
      U(    ;
      L     DB98.DBW  312;
      L     1;
      ==I   ;
      )     ;
      SPBNB _07f;
      L     L#90;
      T     DB98.DBD  360;
_07f: NOP   0;
      U     L      0.0;
      U(    ;
      L     DB98.DBW  312;
      L     2;
      ==I   ;
      )     ;
      SPBNB _080;
      L     L#90;
      T     DB98.DBD  360;
_080: NOP   0;
NETWORK
TITLE =Verifica e Caricamento Impostaz Rotaz Asse B 2 Deposito Box. SX

      U     "MG";
      =     L      0.0;
      U     L      0.0;
      U(    ;
      L     DB98.DBW  316;
      L     0;
      ==I   ;
      )     ;
      SPBNB _081;
      L     L#0;
      T     DB98.DBD  364;
_081: NOP   0;
      U     L      0.0;
      U(    ;
      L     DB98.DBW  316;
      L     1;
      ==I   ;
      )     ;
      SPBNB _082;
      L     L#90;
      T     DB98.DBD  364;
_082: NOP   0;
      U     L      0.0;
      U(    ;
      L     DB98.DBW  316;
      L     2;
      ==I   ;
      )     ;
      SPBNB _083;
      L     L#90;
      T     DB98.DBD  364;
_083: NOP   0;
NETWORK
TITLE =Verifica e Caricamento Impostaz Rotaz Asse B 3 Deposito Box. SX

      U     "MG";
      =     L      0.0;
      U     L      0.0;
      U(    ;
      L     DB98.DBW  320;
      L     0;
      ==I   ;
      )     ;
      SPBNB _084;
      L     L#0;
      T     DB98.DBD  368;
_084: NOP   0;
      U     L      0.0;
      U(    ;
      L     DB98.DBW  320;
      L     1;
      ==I   ;
      )     ;
      SPBNB _085;
      L     L#90;
      T     DB98.DBD  368;
_085: NOP   0;
      U     L      0.0;
      U(    ;
      L     DB98.DBW  320;
      L     2;
      ==I   ;
      )     ;
      SPBNB _086;
      L     L#90;
      T     DB98.DBD  368;
_086: NOP   0;
END_FUNCTION

